|   IBIS Model for tsi109
[IBIS Ver]   3.2
[Disclaimer] This model is subject to change.
   Integrated Device Technology, Inc. ("IDT") hereby grants the
   user of this IBIS model a non-exclusive, nontransferable
   license to use this IBIS model under the following terms. The
   user is granted this license only to use the IBIS model and is
   not granted rights to sell, copy (except as needed to run the
   IBIS model), rent, lease or sub-license the IBIS model in
   whole or in part, or in modified form to anyone. The User may
   modify the IBIS model to suit its specific applications, but
   rights to derivative works and such modifications shall belong
   to IDT. This IBIS model is provided on an AS IS" basis and IDT
   makes absolutely no warranty with respect to the information
   contained herein. IDT DISCLAIMS AND CUSTOMER WAIVES ALL
   WARRANTIES, EXPRESS AND IMPLIED, INCLUDING WARRANTIES OF
   MERCHANTABILITY AND FITNESS FOR A PARTICULAR PURPOSE. THE
   ENTIRE RISK AS TO QUALITY AND PERFORMANCE IS WITH THE USER
   ACCORDINGLY, IN NO EVENT SHALL IDT BE LIABLE FOR ANY DIRECT OR
   INDIRECT DAMAGES, WHETHER IN CONTRACT OR TORT, INCLUDING ANY
   LOST PROFITS OR OTHER INCIDENTAL, CONSEQUENTIAL, EXEMPLARY, OR
   PUNITIVE DAMAGES ARISING OUT OF THE USE OR APPLICATION OF THE
   IBIS model. Further, IDT reserves the right to make changes
   without notice to any product herein to improve reliability,
   function, or design. IDT does not convey any license under
   patent rights or any other intellectual property rights,
   including those of third parties. IDT is not obligated to
   provide maintenance or support for the licensed IBIS model.
[Copyright]   Copyright 2009, Integrated Device Technology, Inc. all
   rights reserved.
[File Name]   tsi109_v3r1_ind.ibs
[File Rev]   3.2
[Date]   03/28/2006
[Notes]
   Revision History
   Rev 1.0
   - 6/17/04 Inital Release. This models is intended for
   evaluation purposes only and does not contain real
   IV/VT curves.  RHB
   Rev 1.1
   - 1/29/2005 First Customer Release. RHB
   Rev 2.0
   -5/24/2005 Regenerated using updated HSPICE models. JMB
   Rev 2.1
   -6/15/2005 Changed models for pins SD_CB[*] to SD_DQ
   from SD_OUT. JMB
   Rev 3.0
   - 02/07/2006  Updated model curves with new simulation data.  RRD
   Rev 3.1
   - 03/28/2006  Add input-only, output-only models.  RRD
   Rev 3.2
   - 09/08/2009 Updated with IDT formatting
[Component] tsi109
[Manufacturer] Integrated Device Technology, Inc.
|   typ   min   max
[Package]
R_pkg   1040.87m   306.00m   1990.00m
L_pkg   5530.5pH   2360.0pH  11100.0pH
C_pkg   2.419pF   1.600pF   4.370pF
[Pin] signal_name   model_name   R_pin   L_pin   C_pin
A1   NC   NC
A2   SD_DQ[56]   SD_DQ   1830.00m  7470.0pH   3.370pF
A3   SD_DQ[60]   SD_DQ   1140.00m  6650.0pH   2.730pF
A4   SD_CLK_N[5]   SD_CLK   1790.00m  6540.0pH   3.670pF
A5   SD_CLK_N[2]   SD_CLK   1690.00m  8020.0pH   2.520pF
A6   SD_CLK_P[2]   SD_CLK   1680.00m  7780.0pH   2.570pF
A7   SD_DQ[34]   SD_DQ   1660.00m  6230.0pH   3.340pF
A8   SD_DQ[38]   SD_DQ   1060.00m  6420.0pH   2.480pF
A9   SD_DQS_P[4]   SD_DQS   1510.00m  7200.0pH   2.400pF
A10   SD_DQS_N[13]   SD_DQS#   1560.00m  6140.0pH   3.180pF
A11   SD_DQ[33]   SD_DQ   1080.00m  6930.0pH   2.450pF
A12   SD_DQ[32]   SD_DQ   1540.00m  6240.0pH   3.020pF
A13   SD_DQ[36]   SD_DQ   1450.00m  5500.0pH   2.910pF
A14   SD_CLK_N[3]   SD_CLK   1530.00m  7950.0pH   2.290pF
A15   SD_CLKFBO_N   SD_OUT   1520.00m  8400.0pH   2.370pF
A16   SD_CLKFBI_P   SD_OUT   1270.00m  4970.0pH   2.770pF
A17   SD_CLK_P[0]   SD_CLK   1520.00m  7380.0pH   2.330pF
A18   SD_DQ[19]   SD_DQ   1030.00m  6390.0pH   2.410pF
A19   SD_DQ[18]   SD_DQ   1000.00m  6450.0pH   2.380pF
A20   SD_DQ[23]   SD_DQ   1020.00m  6410.0pH   2.440pF
A21   SD_DQS_P[2]   SD_DQS   1420.00m  7090.0pH   2.310pF
A22   SD_DQS_N[11]   SD_DQS#   1500.00m  7330.0pH   2.280pF
A23   SD_DQS_P[11]   SD_DQS   1480.00m  7310.0pH   2.390pF
A24   SD_DQ[16]   SD_DQ   1570.00m  6260.0pH   3.010pF
A25   SD_DQ[20]   SD_DQ   1680.00m  6530.0pH   3.200pF
A26   SD_CLK_N[4]   SD_CLK   1700.00m  8530.0pH   2.540pF
A27   SD_CLK_N[1]   SD_CLK   1660.00m  6210.0pH   3.340pF
A28   SD_DQ[3]   SD_DQ   1720.00m  6440.0pH   3.290pF
A29   SD_DQ[2]   SD_DQ   1790.00m  6520.0pH   3.270pF
A30   SD_DQ[6]   SD_DQ   1750.00m  11100.0pH  2.260pF
A31   SD_DQS_N[0]   SD_DQS#   1770.00m  7880.0pH   2.650pF
A32   VSS_IO   GND
B1   SD_DQS_P[16]   SD_DQS   1750.00m  7110.0pH   3.440pF
B2   SD_DQ[57]   SD_DQ   1140.00m  6410.0pH   2.660pF
B3   VSS_IO   GND
B4   NC   NC
B5   SD_CLK_P[5]   SD_CLK   1800.00m  6730.0pH   3.560pF
B6   VSS_IO   GND
B7   SD_DQ[35]   SD_DQ   1590.00m  6010.0pH   3.050pF
B8   SD_DQ[39]   SD_DQ   1030.00m  6400.0pH   2.510pF
B9   VSS_IO   GND
B10   SD_DQS_N[4]   SD_DQS#   1530.00m  7070.0pH   2.410pF
B11   SD_DQS_P[13]   SD_DQS   1560.00m  6020.0pH   3.250pF
B12   VSS_IO   GND
B13   SD_DQ[37]   SD_DQ   964.00m   6360.0pH   2.410pF
B14   SD_CLK_P[3]   SD_CLK   1530.00m  7890.0pH   2.390pF
B15   VSS_IO   GND
B16   SD_CLKFBO_P   SD_OUT   1510.00m  8250.0pH   2.380pF
B17   SD_CLKFBI_N   SD_OUT   1270.00m  5580.0pH   2.860pF
B18   SD_CLK_N[0]   SD_CLK   1500.00m  7590.0pH   2.420pF
B19   VSS_IO   GND
B20   SD_DQ[22]   SD_DQ   1080.00m  7000.0pH   2.540pF
B21   SD_DQS_N[2]   SD_DQS#   1450.00m  7330.0pH   2.340pF
B22   VSS_IO   GND
B23   SD_DQ[17]   SD_DQ   1070.00m  6980.0pH   2.470pF
B24   SD_DQ[21]   SD_DQ   1110.00m  6950.0pH   2.500pF
B25   VSS_IO   GND
B26   SD_CLK_P[4]   SD_CLK   1710.00m  8340.0pH   2.600pF
B27   SD_CLK_P[1]   SD_CLK   1630.00m  6310.0pH   3.440pF
B28   VSS_IO   GND
B29   SD_DQ[7]   SD_DQ   1560.00m  7000.0pH   3.180pF
B30   SD_DQS_P[0]   SD_DQS   1770.00m  8010.0pH   2.710pF
B31   VSS_IO   GND
B32   SD_DQS_N[9]   SD_DQS#   1740.00m  8460.0pH   2.590pF
C1   VSS_IO   GND
C2   SD_DQS_N[16]   SD_DQS#   1730.00m  6400.0pH   3.630pF
C3   SD_DQ[61]   SD_DQ   1200.00m  7870.0pH   2.680pF
C4   VDD_SD   POWER
C5   SD_DQ[54]   SD_DQ   1540.00m  5890.0pH   3.090pF
C6   SD_DQS_N[6]   SD_DQS#   1420.00m  7180.0pH   2.350pF
C7   VDD_SD   POWER
C8   SD_DQ[53]   SD_DQ   1370.00m  5230.0pH   2.990pF
C9   SD_DQ[43]   SD_DQ   1380.00m  5690.0pH   2.850pF
C10   VDD_SD   POWER
C11   SD_DQS_N[5]   SD_DQS#   1220.00m  4990.0pH   2.770pF
C12   SD_DQS_P[14]   SD_DQS   1200.00m  6340.0pH   2.120pF
C13   VDD_SD   POWER
C14   SD_CB[3]   SD_DQ   812.00m   5540.0pH   2.170pF
C15   SD_CB[6]   SD_DQ   789.00m   5680.0pH   2.170pF
C16   VDD_SD   POWER
C17   NC   NC
C18   VDD_SD   POWER
C19   SD_CB[5]   SD_DQ   811.00m   5770.0pH   2.160pF
C20   SD_DQ[26]   SD_DQ   1140.00m  5190.0pH   2.610pF
C21   VDD_SD   POWER
C22   SD_DQS_N[12]   SD_DQS#   1250.00m  5070.0pH   2.780pF
C23   NC   NC
C24   VDD_SD   POWER
C25   SD_DQ[11]   SD_DQ   1030.00m  7050.0pH   2.450pF
C26   SD_DQ[15]   SD_DQ   1330.00m  5270.0pH   2.780pF
C27   VDD_SD   POWER
C28   NC   NC
C29   VDD_SD   POWER
C30   NC   NC
C31   SD_DQS_P[9]   SD_DQS   1720.00m  8030.0pH   2.610pF
C32   SD_DQ[1]   SD_DQ   1780.00m  6690.0pH   3.520pF
D1   SD_DQS_P[7]   SD_DQS   1620.00m  7470.0pH   2.530pF
D2   SD_DQS_N[7]   SD_DQS#   1670.00m  8310.0pH   2.620pF
D3   SD_DQ[62]   SD_DQ   1490.00m  6280.0pH   2.940pF
D4   SD_DQ[51]   SD_DQ   1520.00m  6140.0pH   3.220pF
D5   SD_DQ[55]   SD_DQ   1470.00m  6410.0pH   2.940pF
D6   SD_DQS_P[6]   SD_DQS   1430.00m  7550.0pH   2.330pF
D7   SD_DQS_P[15]   SD_DQS   1320.00m  5410.0pH   2.860pF
D8   SD_DQ[48]   SD_DQ   962.00m   6180.0pH   2.360pF
D9   SD_DQ[52]   SD_DQ   924.00m   6060.0pH   2.270pF
D10   SD_DQ[47]   SD_DQ   1220.00m  5520.0pH   2.700pF
D11   SD_DQS_P[5]   SD_DQS   1220.00m  5110.0pH   2.760pF
D12   SD_DQS_N[14]   SD_DQS#   1200.00m  6280.0pH   2.110pF
D13   SD_DQ[40]   SD_DQ   1150.00m  5330.0pH   2.620pF
D14   SD_DQ[44]   SD_DQ   890.00m   6610.0pH   2.280pF
D15   SD_CB[7]   SD_DQ   670.00m   4800.0pH   2.030pF
D16   SD_DQS_N[8]   SD_DQS#   987.00m   5460.0pH   2.040pF
D17   SD_DQS_N[17]   SD_DQS#   1040.00m  6330.0pH   2.120pF
D18   SD_CB[1]   SD_DQ   1140.00m  5740.0pH   2.500pF
D19   SD_CB[4]   SD_DQ   1120.00m  4840.0pH   2.630pF
D20   SD_DQ[31]   SD_DQ   808.00m   5620.0pH   2.150pF
D21   SD_DQS_P[3]   SD_DQS   1210.00m  5190.0pH   2.790pF
D22   SD_DQS_P[12]   SD_DQS   1250.00m  5470.0pH   2.910pF
D23   SD_DQ[25]   SD_DQ   1230.00m  5240.0pH   2.570pF
D24   SD_DQ[29]   SD_DQ   1230.00m  5420.0pH   2.890pF
D25   SD_DQ[10]   SD_DQ   1020.00m  6620.0pH   2.390pF
D26   SD_DQ[14]   SD_DQ   982.00m   6140.0pH   2.300pF
D27   SD_DQS_N[1]   SD_DQS#   1370.00m  7580.0pH   2.280pF
D28   SD_DQS_P[10]   SD_DQS   1370.00m  5580.0pH   2.950pF
D29   SD_DQ[8]   SD_DQ   1560.00m  6180.0pH   3.040pF
D30   NC   NC
D31   SD_DQ[0]   SD_DQ   1660.00m  6770.0pH   3.180pF
D32   SD_DQ[5]   SD_DQ   1760.00m  6720.0pH   3.460pF
E1   SD_DQ[63]   SD_DQ   1670.00m  6670.0pH   3.160pF
E2   SD_DQ[58]   SD_DQ   1560.00m  6080.0pH   3.120pF
E3   VSS_IO   GND
E4   NC   NC
E5   SD_DQ[50]   SD_DQ   1460.00m  6250.0pH   2.860pF
E6   VSS_IO   GND
E7   SD_DQS_N[15]   SD_DQS#   1320.00m  5370.0pH   2.900pF
E8   SD_DQ[49]   SD_DQ   1150.00m  5080.0pH   2.550pF
E9   VSS_IO   GND
E10   SD_DQ[42]   SD_DQ   777.00m   5310.0pH   2.020pF
E11   SD_DQ[46]   SD_DQ   737.00m   5600.0pH   2.030pF
E12   VSS_IO   GND
E13   SD_DQ[41]   SD_DQ   1010.00m  4810.0pH   2.320pF
E14   SD_DQ[45]   SD_DQ   841.00m   6000.0pH   2.200pF
E15   VSS_IO   GND
E16   SD_DQS_P[8]   SD_DQS   966.00m   5460.0pH   1.970pF
E17   SD_DQS_P[17]   SD_DQS   1050.00m  6280.0pH   2.050pF
E18   SD_CB[0]   SD_DQ   605.00m   4680.0pH   1.880pF
E19   VSS_IO   GND
E20   SD_DQ[30]   SD_DQ   1000.00m  4730.0pH   2.250pF
E21   SD_DQS_N[3]   SD_DQS#   1220.00m  5610.0pH   2.800pF
E22   VSS_IO   GND
E23   SD_DQ[24]   SD_DQ   1110.00m  5050.0pH   2.490pF
E24   SD_DQ[28]   SD_DQ   1230.00m  5670.0pH   2.600pF
E25   VSS_IO   GND
E26   SD_DQS_P[1]   SD_DQS   1370.00m  8240.0pH   2.290pF
E27   SD_DQS_N[10]   SD_DQS#   1350.00m  5470.0pH   3.060pF
E28   VDD_SD   POWER
E29   SD_DQ[13]   SD_DQ   1290.00m  5480.0pH   2.860pF
E30   VSS_IO   GND
E31   SD_DQ[4]   SD_DQ   1560.00m  6390.0pH   3.020pF
E32   CG_PB_SELECT[1]   GEN18_IN   1090.00m  6830.0pH   2.480pF
F1   SD_DQ[59]   SD_DQ   1630.00m  6800.0pH   3.100pF
F2   VSS_IO   GND
F3   NC   NC
F4   NC   NC
F5   NC   NC
F6   NC   NC
F7   SD_ODT[3]   SD_OUT   732.00m   5070.0pH   2.050pF
F8   NC   NC
F9   SD_CSn[1]   SD_OUT   1100.00m  5310.0pH   2.390pF
F10   VDD_SD   POWER
F11   SD_ODT[0]   SD_OUT   592.00m   4280.0pH   1.960pF
F12   NC   NC
F13   VDD_SD   POWER
F14   SD_RASn   SD_OUT   821.00m   4190.0pH   2.230pF
F15   SD_CB[2]   SD_DQ   929.00m   4810.0pH   2.220pF
F16   SD_DLL_TEST[0]   SD_OUT   820.00m   4110.0pH   2.060pF
F17   VDD_SD   POWER
F18   SD_DLL_TEST[1]   SD_OUT   872.00m   4480.0pH   2.170pF
F19   SD_DQ[27]   SD_DQ   647.00m   4860.0pH   1.920pF
F20   SD_A[6]   SD_OUT   919.00m   4540.0pH   2.310pF
F21   VDD_SD   POWER
F22   SD_VREF[1]   POWER   944.00m   4570.0pH   2.260pF
F23   SD_BA[2]   SD_OUT   732.00m   5230.0pH   1.970pF
F24   VDD_SD   POWER
F25   NC   NC
F26   SD_CLKEN[1]   SD_OUT   1140.00m  4900.0pH   2.470pF
F27   VSS_IO   GND
F28   SD_DQ[9]   SD_DQ   1320.00m  5560.0pH   3.000pF
F29   SD_DQ[12]   SD_DQ   1390.00m  5930.0pH   2.860pF
F30   PB_A[33]   PB_IO   1420.00m  5680.0pH   2.910pF
F31   PB_RSTn   GEN18_OUT   981.00m   5810.0pH   2.480pF
F32   CG_REF   GEN18_IN   1050.00m  6430.0pH   2.500pF
G1   HLP_AD[0]   GEN33_IO_tf06it0nn2  1030.00m  6280.0pH   2.530pF
G2   HLP_AD[1]   GEN33_IO_tf06it0nn2  1290.00m  5250.0pH   2.780pF
G3   SD_I2C_CLK   GEN33_OUT_tf12it0pu2 1320.00m  5560.0pH   2.720pF
G4   SD_I2C_SD   GEN33_IO_tf12it0pu2  1200.00m  5350.0pH   2.530pF
G5   HLP_AD[8]   GEN33_IO_tf06it0nn2  1300.00m  5630.0pH   2.620pF
G6   HLP_AD[9]   GEN33_IO_tf06it0nn2  1100.00m  4780.0pH   2.350pF
G7   VSS_IO   GND
G8   SD_ODT[1]   SD_OUT   846.00m   4100.0pH   2.080pF
G9   SD_CSn[3]   SD_OUT   1010.00m  5160.0pH   2.230pF
G10   SD_A[13]   SD_OUT   638.00m   5140.0pH   1.970pF
G11   SD_ODT[2]   SD_OUT   868.00m   4580.0pH   2.050pF
G12   SD_CASn   SD_OUT   821.00m   4410.0pH   2.070pF
G13   SD_WEn   SD_OUT   614.00m   5160.0pH   1.830pF
G14   SD_CSn[0]   SD_OUT   817.00m   4790.0pH   2.120pF
G15   SD_A[10]   SD_OUT   747.00m   3920.0pH   2.090pF
G16   SD_A[0]   SD_OUT   780.00m   4450.0pH   2.130pF
G17   SD_A[2]   SD_OUT   826.00m   4910.0pH   2.100pF
G18   SD_A[1]   SD_OUT   833.00m   4310.0pH   2.050pF
G19   SD_A[4]   SD_OUT   711.00m   6210.0pH   2.120pF
G20   SD_A[9]   SD_OUT   860.00m   5070.0pH   2.160pF
G21   SD_A[8]   SD_OUT   623.00m   5260.0pH   1.830pF
G22   SD_A[11]   SD_OUT   603.00m   4440.0pH   1.830pF
G23   SD_A[14]   SD_OUT   600.00m   4560.0pH   1.860pF
G24   SD_A[15]   SD_OUT   575.00m   4280.0pH   1.840pF
G25   SD_CLKEN[0]   SD_OUT   939.00m   4550.0pH   2.420pF
G26   VDD_SD   POWER
G27   NC   NC
G28   VSS_IO   GND
G29   CG_SD_SELECT[0]   GEN18_IN   814.00m   5410.0pH   2.190pF
G30   NC   NC
G31   VSS_IO   GND
G32   CG_SD_SELECT[1]   GEN18_IN   1370.00m  5250.0pH   2.920pF
H1   HLP_AD[2]   GEN33_IO_tf06it0nn2  996.00m   6180.0pH   2.390pF
H2   HLP_AD[3]   GEN33_IO_tf06it0nn2  1260.00m  5200.0pH   2.750pF
H3   HLP_AD[4]   GEN33_IO_tf06it0nn2  837.00m   5550.0pH   2.280pF
H4   VSS_IO   GND
H5   HLP_AD[5]   GEN33_IO_tf06it0nn2  1130.00m  4790.0pH   2.460pF
H6   HLP_AD[6]   GEN33_IO_tf06it0nn2  870.00m   6390.0pH   2.250pF
H7   HLP_AD[7]   GEN33_IO_tf06it0nn2  853.00m   4190.0pH   2.180pF
H8   NC   NC
H9   VSS_IO   GND
H10   VDD_SD   POWER
H11   VDD_SD   POWER
H12   SD_VREF[0]   POWER   610.00m   3730.0pH   1.830pF
H13   VSS_IO   GND
H14   SD_CSn[2]   SD_OUT   649.00m   8400.0pH   1.970pF
H15   SD_BA[0]   SD_OUT   961.00m   4300.0pH   2.370pF
H16   SD_BA[1]   SD_OUT   736.00m   6940.0pH   2.100pF
H17   VSS_IO   GND
H18   SD_A[3]   SD_OUT   751.00m   4280.0pH   1.920pF
H19   SD_A[5]   SD_OUT   862.00m   5240.0pH   2.080pF
H20   VSS_IO   GND
H21   SD_A[7]   SD_OUT   569.00m   4850.0pH   1.740pF
H22   SD_A[12]   SD_OUT   901.00m   4490.0pH   2.160pF
H23   VDD_SD   POWER
H24   VDD_SD   POWER
H25   VSS_IO   GND
H26   PB_A[34]   PB_IO   960.00m   4820.0pH   2.220pF
H27   VDD_PB   POWER
H28   CG_SD_SELECT[2]   GEN18_IN   684.00m   4920.0pH   2.040pF
H29   CG_PB_SELECT[2]   GEN18_IN   758.00m   5350.0pH   2.080pF
H30   VDD_PB   POWER
H31   CG_PB_CLKO[1]   GEN18_OUT   923.00m   6270.0pH   2.370pF
H32   CG_PB_CLKO[0]   GEN18_OUT   971.00m   6200.0pH   2.410pF
J1   CLKGEN_PLL_AVDD[1]   POWER   491.00m   4760.0pH   3.100pF
J2   CLKGEN_PLL_AVSS[1]   POWER   430.00m   3090.0pH   4.370pF
J3   HLP_AD[10]   GEN33_IO_tf06it0nn2  904.00m   5880.0pH   2.270pF
J4   HLP_AD[11]   GEN33_IO_tf06it0nn2  749.00m   5350.0pH   2.120pF
J5   HLP_AD[12]   GEN33_IO_tf06it0nn2  698.00m   5380.0pH   1.950pF
J6   HLP_AD[13]   GEN33_IO_tf06it0nn2  684.00m   5640.0pH   1.990pF
J7   HLP_AD[14]   GEN33_IO_tf06it0nn2  961.00m   6170.0pH   2.390pF
J8   HLP_AD[15]   GEN33_IO_tf06it0nn2  925.00m   4660.0pH   2.160pF
J9   VDD_PC   POWER
J10   VSS_IO   GND
J11   VDD_SD   POWER
J12   VSS_IO   GND
J13   VDD_SD   POWER
J14   VSS_IO   GND
J15   VDD_SD   POWER
J16   VSS_IO   GND
J17   VDD_SD   POWER
J18   VSS_IO   GND
J19   VDD_SD   POWER
J20   VSS_IO   GND
J21   VDD_SD   POWER
J22   VSS_IO   GND
J23   VDD_SD   POWER
J24   VSS_IO   GND
J25   PB_A[35]   PB_IO   802.00m   4510.0pH   2.010pF
J26   PB_A[10]   PB_IO   903.00m   4680.0pH   2.070pF
J27   PB_A[32]   PB_IO   1000.00m  4980.0pH   2.290pF
J28   PB_A[0]   PB_IO   1040.00m  4790.0pH   2.360pF
J29   PB_TSIZ[2]   PB_IO   839.00m   5660.0pH   2.180pF
J30   NC   NC
J31   CG_PB_SELECT[0]   GEN18_IN   965.00m   6110.0pH   2.420pF
J32   CG_PB_CLKO[2]   GEN18_OUT   977.00m   5900.0pH   2.420pF
K1   HLP_AD[16]   GEN33_IO_tf06it0nn2  1040.00m  6310.0pH   2.480pF
K2   VSS_IO   GND
K3   HLP_AD[17]   GEN33_IO_tf06it0nn2  811.00m   5330.0pH   2.190pF
K4   HLP_AD[18]   GEN33_IO_tf06it0nn2  730.00m   5200.0pH   2.080pF
K5   HLP_AD[19]   GEN33_IO_tf06it0nn2  689.00m   4660.0pH   2.040pF
K6   HLP_AD[20]   GEN33_IO_tf06it0nn2  839.00m   5820.0pH   2.220pF
K7   VSS_IO   GND
K8   HLP_AD[21]   GEN33_IO_tf06it0nn2  923.00m   4970.0pH   2.600pF
K9   VDD_PC   POWER
K10   VDD_PC   POWER
K11   VSS_IO   GND
K12   VDD_SD   POWER
K13   VDD_SD   POWER
K14   VDD_SD   POWER
K15   VDD_SD   POWER
K16   VDD_SD   POWER
K17   VDD_SD   POWER
K18   VDD_SD   POWER
K19   VDD_SD   POWER
K20   VDD_SD   POWER
K21   VDD_SD   POWER
K22   VDD_SD   POWER
K23   VSS_IO   GND
K24   VDD_PB   POWER
K25   PB_TT[3]   PB_IO   1140.00m  5840.0pH   2.280pF
K26   PB_A[8]   PB_IO   739.00m   6390.0pH   2.000pF
K27   PB_A[6]   PB_IO   983.00m   4960.0pH   2.270pF
K28   VSS_IO   GND
K29   CLKGEN_PLL_AVDD[0]   POWER   321.00m   2490.0pH   3.650pF
K30   CLKGEN_PLL_AVSS[0]   POWER   444.00m   4160.0pH   2.900pF
K31   VSS_IO   GND
K32   PB_A[4]   PB_IO   954.00m   5740.0pH   2.420pF
L1   HLP_AD[22]   GEN33_IO_tf06it0nn2  934.00m   5910.0pH   2.300pF
L2   HLP_AD[23]   GEN33_IO_tf06it0nn2  1260.00m  5350.0pH   2.610pF
L3   HLP_AD[24]   GEN33_IO_tf06it0nn2  788.00m   5570.0pH   2.150pF
L4   HLP_AD[25]   GEN33_IO_tf06it0nn2  1030.00m  4620.0pH   2.370pF
L5   VSS_IO   GND
L6   HLP_AD[26]   GEN33_IO_tf06it0nn2  897.00m   4290.0pH   2.260pF
L7   HLP_AD[27]   GEN33_IO_tf06it0nn2  750.00m   6430.0pH   1.890pF
L8   HLP_AD[28]   GEN33_IO_tf06it0nn2  877.00m   4660.0pH   2.060pF
L9   VDD_PC   POWER
L10   VDD_PC   POWER
L11   VSS_IO   GND
L12   VSS_IO   GND
L13   VSS_IO   GND
L14   VSS_IO   GND
L15   VSS_IO   GND
L16   VSS_IO   GND
L17   VSS_IO   GND
L18   VSS_IO   GND
L19   VSS_IO   GND
L20   VSS_IO   GND
L21   VSS_IO   GND
L22   VSS_IO   GND
L23   VDD_PB   POWER
L24   VDD_PB   POWER
L25   PB_AP[4]   PB_IO   753.00m   7660.0pH   2.170pF
L26   PB_TT[1]   PB_IO   315.00m   3030.0pH   2.770pF
L27   VDD_PB   POWER
L28   PB_TT[0]   PB_IO   649.00m   4750.0pH   1.970pF
L29   PB_TT[4]   PB_IO   722.00m   5540.0pH   2.110pF
L30   VDD_PB   POWER
L31   SD_PLL_AVDD   POWER   488.00m   4020.0pH   2.960pF
L32   SD_PLL_AVSS   POWER   386.00m   2570.0pH   4.370pF
M1   HLP_WEn   GEN33_OUT_tf06it0nn2 983.00m   6520.0pH   2.420pF
M2   HLP_CSn[0]   GEN33_OUT_tf06it0nn2 1350.00m  5870.0pH   2.700pF
M3   HLP_CSn[2]   GEN33_OUT_tf06it0nn2 1190.00m  5000.0pH   2.760pF
M4   HLP_CSn[3]   GEN33_OUT_tf06it0nn2 1010.00m  4430.0pH   2.390pF
M5   HLP_LE   GEN33_OUT_tf06it0nn2 1030.00m  5260.0pH   2.300pF
M6   HLP_AD[29]   GEN33_IO_tf06it0nn2  843.00m   3830.0pH   2.240pF
M7   HLP_AD[30]   GEN33_IO_tf06it0nn2  770.00m   5580.0pH   1.970pF
M8   HLP_AD[31]   GEN33_IO_tf06it0nn2  811.00m   4290.0pH   1.990pF
M9   VDD_PC   POWER
M10   VDD_PC   POWER
M11   VSS_IO   GND
M12   VSS   GND
M13   VDD   POWER
M14   VSS   GND
M15   VDD   POWER
M16   VSS   GND
M17   VDD   POWER
M18   VSS   GND
M19   VDD   POWER
M20   VSS   GND
M21   VDD   POWER
M22   VSS_IO   GND
M23   VDD_PB   POWER
M24   VSS_IO   GND
M25   PB_INTn[1]   PB_OUT   1040.00m  5240.0pH   2.930pF
M26   PB_INTn[2]   PB_OUT   890.00m   4640.0pH   2.040pF
M27   PB_INTn[3]   PB_OUT   912.00m   4540.0pH   2.110pF
M28   PB_A[2]   PB_IO   953.00m   4290.0pH   2.310pF
M29   PB_PLL_AVSS   POWER   306.00m   2360.0pH   3.640pF
M30   PB_PLL_AVDD   POWER   1220.00m  5280.0pH   2.510pF
M31   PB_TSIZ[1]   PB_IO   867.00m   5610.0pH   2.270pF
M32   SD_SYSCLK   GEN18_IN   917.00m   5720.0pH   2.310pF
N1   HLP_CSn[1]   GEN33_OUT_tf06it0nn2 978.00m   5920.0pH   2.390pF
N2   VSS_IO   GND
N3   HLP_RDYn   GEN33_IN_it2nn2   752.00m   4880.0pH   2.120pF
N4   HLP_OEn   GEN33_OUT_tf06it0nn2 1090.00m  4980.0pH   2.430pF
N5   GPIO[0]   GEN33_IO_tf06it0nn2  807.00m   5660.0pH   2.090pF
N6   GPIO[1]   GEN33_IO_tf06it0nn2  866.00m   4180.0pH   2.100pF
N7   VSS_IO   GND
N8   U_1_RX   GEN33_IN_it2nn2   627.00m   3560.0pH   1.820pF
N9   VDD_PC   POWER
N10   VDD_PC   POWER
N11   VSS_IO   GND
N12   VDD   POWER
N13   VSS   GND
N14   VDD   POWER
N15   VSS   GND
N16   VDD   POWER
N17   VSS   GND
N18   VDD   POWER
N19   VSS   GND
N20   VDD   POWER
N21   VSS   GND
N22   VSS_IO   GND
N23   VDD_PB   POWER
N24   VDD_PB   POWER
N25   VSS_IO   GND
N26   PB_HITn[1]   PB_IN   946.00m   4810.0pH   2.110pF
N27   PB_BRn[1]   PB_IN   834.00m   4400.0pH   2.030pF
N28   VSS_IO   GND
N29   PB_BRn[0]   PB_IN   676.00m   4760.0pH   1.960pF
N30   PB_AP[2]   PB_IO   823.00m   5440.0pH   2.240pF
N31   VSS_IO   GND
N32   PB_AP[3]   PB_IO   1370.00m  5330.0pH   2.930pF
P1   JTAG_TDO   GEN33_OUT_tf02it0nn2 875.00m   5320.0pH   2.270pF
P2   JTAG_TDI   GEN33_IN_it2pu2   1220.00m  4910.0pH   2.750pF
P3   GPIO[2]   GEN33_IO_tf06it0nn2  730.00m   5170.0pH   2.130pF
P4   VSS_IO   GND
P5   GPIO[3]   GEN33_IO_tf06it0nn2  708.00m   5120.0pH   1.950pF
P6   GPIO[4]   GEN33_IO_tf06it0nn2  876.00m   4260.0pH   2.400pF
P7   GPIO[5]   GEN33_IO_tf06it0nn2  837.00m   6940.0pH   2.070pF
P8   U_0_RX   GEN33_IN_it2nn2   533.00m   3260.0pH   1.750pF
P9   VDD_PC   POWER
P10   VDD_PC   POWER
P11   VSS_IO   GND
P12   VSS   GND
P13   VDD   POWER
P14   VSS   GND
P15   VDD   POWER
P16   VSS   GND
P17   VDD   POWER
P18   VSS   GND
P19   VDD   POWER
P20   VSS   GND
P21   VDD   POWER
P22   VSS_IO   GND
P23   VDD_PB   POWER
P24   VSS_IO   GND
P25   PB_AP[0]   PB_IO   815.00m   4350.0pH   1.940pF
P26   PB_TSIZ[0]   PB_IO   696.00m   5530.0pH   2.040pF
P27   VDD_PB   POWER
P28   PB_TT[2]   PB_IO   659.00m   4860.0pH   1.860pF
P29   PB_QACKn[1]   PB_OUT   741.00m   5010.0pH   2.130pF
P30   VDD_PB   POWER
P31   PB_TBSTn   PB_IO   1230.00m  5310.0pH   2.520pF
P32   PB_SYSCLK   PB_IN   900.00m   6160.0pH   2.320pF
R1   TEST_TM[1]   GEN33_IO_tf02it0nn2  955.00m   5990.0pH   2.330pF
R2   JTAG_TCK   GEN33_IN_it2pu2   1220.00m  5440.0pH   2.730pF
R3   GPIO[6]   GEN33_IO_tf06it0nn2  721.00m   5020.0pH   2.000pF
R4   INT[0]   GEN33_IN_it2nn2   726.00m   5300.0pH   2.040pF
R5   GPIO[7]   GEN33_IO_tf06it0nn2  842.00m   4090.0pH   2.240pF
R6   GPIO[8]   GEN33_IO_tf06it0nn2  833.00m   4360.0pH   2.060pF
R7   GPIO[9]   GEN33_IO_tf06it0nn2  913.00m   4860.0pH   2.080pF
R8   U_1_TX   GEN33_OUT_tf06it0nn2 606.00m   3210.0pH   1.800pF
R9   VDD_PC   POWER
R10   VDD_PC   POWER
R11   VSS_IO   GND
R12   VDD   POWER
R13   VSS   GND
R14   VDD   POWER
R15   VSS   GND
R16   VDD   POWER
R17   VSS   GND
R18   VDD   POWER
R19   VSS   GND
R20   VDD   POWER
R21   VSS   GND
R22   VSS_IO   GND
R23   VDD_PB   POWER
R24   VDD_PB   POWER
R25   PB_QACKn[0]   PB_OUT   647.00m   6420.0pH   1.690pF
R26   PB_A[14]   PB_IO   713.00m   6620.0pH   1.930pF
R27   PB_A[23]   PB_IO   805.00m   4400.0pH   2.000pF
R28   PB_GBLn   PB_IO   924.00m   4510.0pH   2.140pF
R29   PB_A[7]   PB_IO   715.00m   5430.0pH   2.110pF
R30   PB_A[9]   PB_IO   1120.00m  4880.0pH   2.400pF
R31   PB_AP[1]   PB_IO   1200.00m  5610.0pH   2.520pF
R32   PB_HITn[0]   PB_IN   1320.00m  5290.0pH   2.870pF
T1   TEST_TM[3]   GEN33_IO_tf02it0nn2  1310.00m  5340.0pH   2.700pF
T2   VSS_IO   GND
T3   JTAG_TRSTn   GEN33_IN_it2pu2   1120.00m  5010.0pH   2.430pF
T4   GPIO[10]   GEN33_IO_tf06it0nn2  959.00m   5830.0pH   2.390pF
T5   GPIO[11]   GEN33_IO_tf06it0nn2  911.00m   4960.0pH   2.190pF
T6   INT[2]   GEN33_IN_it2nn2   884.00m   7680.0pH   2.250pF
T7   VSS_IO   GND
T8   U_0_TX   GEN33_OUT_tf06it0nn2 494.00m   3200.0pH   1.630pF
T9   VDD_PC   POWER
T10   VDD_PC   POWER
T11   VSS_IO   GND
T12   VSS   GND
T13   VDD   POWER
T14   VSS   GND
T15   VDD   POWER
T16   VSS   GND
T17   VDD   POWER
T18   VSS   GND
T19   VDD   POWER
T20   VSS   GND
T21   VDD   POWER
T22   VSS_IO   GND
T23   VDD_PB   POWER
T24   VSS_IO   GND
T25   PB_A[24]   PB_IO   674.00m   5920.0pH   2.010pF
T26   PB_A[16]   PB_IO   690.00m   5100.0pH   1.950pF
T27   PB_A[3]   PB_IO   856.00m   4060.0pH   2.110pF
T28   VSS_IO   GND
T29   PB_A[1]   PB_IO   714.00m   4980.0pH   1.970pF
T30   PB_A[12]   PB_IO   998.00m   3970.0pH   2.400pF
T31   VSS_IO   GND
T32   PB_INTn[0]   PB_OUT   909.00m   5820.0pH   2.290pF
U1   TEST_TM[2]   GEN33_IO_tf02it0nn2  906.00m   5850.0pH   2.260pF
U2   JTAG_TMS   GEN33_IN_it2pu2   1140.00m  4560.0pH   2.660pF
U3   TEST_ON   GEN33_IN_it2pd2   1030.00m  4240.0pH   2.510pF
U4   INT[1]   GEN33_IN_it2nn2   778.00m   5530.0pH   2.060pF
U5   VSS_IO   GND
U6   GPIO[12]   GEN33_IO_tf06it0nn2  856.00m   4770.0pH   2.110pF
U7   GPIO[13]   GEN33_IO_tf06it0nn2  755.00m   5630.0pH   2.000pF
U8   I2C_SCLK   GEN33_OUT_tf12it0nn2 510.00m   3290.0pH   1.600pF
U9   VDD_PC   POWER
U10   VDD_PC   POWER
U11   VSS_IO   GND
U12   VDD   POWER
U13   VSS   GND
U14   VDD   POWER
U15   VSS   GND
U16   VDD   POWER
U17   VSS   GND
U18   VDD   POWER
U19   VSS   GND
U20   VDD   POWER
U21   VSS   GND
U22   VSS_IO   GND
U23   VDD_PB   POWER
U24   VDD_PB   POWER
U25   VSS_IO   GND
U26   PB_TSn   PB_IO   647.00m   5230.0pH   1.900pF
U27   VDD_PB   POWER
U28   PB_A[21]   PB_IO   891.00m   4330.0pH   2.190pF
U29   PB_DTI[0]   PB_OUT   1050.00m  5060.0pH   2.310pF
U30   VDD_PB   POWER
U31   PB_A[20]   PB_IO   772.00m   5200.0pH   2.180pF
U32   PB_TAn   PB_OUT   1340.00m  5580.0pH   2.720pF
V1   TEST_TM[0]   GEN33_IO_tf02it0nn2  876.00m   5600.0pH   2.220pF
V2   TEST_BIDR_CTL   GEN33_IN_it2pd2   794.00m   5170.0pH   2.170pF
V3   OCN_RSTn   GEN33_IN_it2nn2   785.00m   5110.0pH   2.170pF
V4   GPIO[14]   GEN33_IO_tf06it0nn2  733.00m   6010.0pH   2.010pF
V5   GPIO[15]   GEN33_IO_tf06it0nn2  751.00m   6450.0pH   1.870pF
V6   INT[3]   GEN33_IN_it2nn2   836.00m   3970.0pH   2.080pF
V7   NC   NC
V8   I2C_SD   GEN33_IO_tf12it0nn2  608.00m   3400.0pH   1.860pF
V9   VDD_PC   POWER
V10   VDD_PC   POWER
V11   VSS_IO   GND
V12   VSS   GND
V13   VDD   POWER
V14   VSS   GND
V15   VDD   POWER
V16   VSS   GND
V17   VDD   POWER
V18   VSS   GND
V19   VDD   POWER
V20   VSS   GND
V21   VDD   POWER
V22   VSS_IO   GND
V23   VDD_PB   POWER
V24   VSS_IO   GND
V25   PB_TEAn   PB_OUT   672.00m   6090.0pH   1.860pF
V26   PB_A[22]   PB_IO   836.00m   4100.0pH   2.040pF
V27   PB_A[18]   PB_IO   764.00m   5560.0pH   2.170pF
V28   PB_BGn[1]   PB_OUT   944.00m   4630.0pH   2.130pF
V29   PB_BGn[0]   PB_OUT   739.00m   4930.0pH   2.050pF
V30   PB_A[5]   PB_IO   736.00m   4980.0pH   2.100pF
V31   PB_A[13]   PB_IO   874.00m   5700.0pH   2.290pF
V32   PB_RSTOD   PB_IN   1350.00m  5580.0pH   2.940pF
W1   E_MDIO   GEN33_IO_tf12it0nn2  880.00m   5470.0pH   2.250pF
W2   VSS_IO   GND
W3   E_MDC   GEN33_OUT_tf12it0nn2 1300.00m  5740.0pH   2.690pF
W4   E_1_TCG[9]   GEN33_OUT_tf12it0nn2 665.00m   4520.0pH   1.950pF
W5   E_0_TCG[9]   GEN33_OUT_tf12it0nn2 1180.00m  5540.0pH   2.440pF
W6   E_0_TCG[8]   GEN33_OUT_tf12it0nn2 741.00m   5690.0pH   2.110pF
W7   VSS_IO   GND
W8   E_0_TCG[7]   GEN33_OUT_tf12it0nn2 879.00m   5210.0pH   2.000pF
W9   VDD_PC   POWER
W10   VDD_PC   POWER
W11   VSS_IO   GND
W12   VDD   POWER
W13   VSS   GND
W14   VDD   POWER
W15   VSS   GND
W16   VDD   POWER
W17   VSS   GND
W18   VDD   POWER
W19   VSS   GND
W20   VDD   POWER
W21   VSS   GND
W22   VSS_IO   GND
W23   VDD_PB   POWER
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|**********************DIFF PIN*************************************************
[Diff_pin] inv_pin vdiff tdelay_typ tdelay_min tdelay_max |Signal Comp Signal
A16   B17   .250V   0ns   NA   NA  |SD_CLKFBI_P   SD_CLKFBI_N
B16   A15   .250V   0ns   NA   NA  |SD_CLKFBO_P   SD_CLKFBO_N
A17   B18   .250V   0ns   NA   NA  |SD_CLK_P[0]   SD_CLK_N[0]
B27   A27   .250V   0ns   NA   NA  |SD_CLK_P[1]   SD_CLK_N[1]
A6   A5   .250V   0ns   NA   NA  |SD_CLK_P[2]   SD_CLK_N[2]
B14   A14   .250V   0ns   NA   NA  |SD_CLK_P[3]   SD_CLK_N[3]
B26   A26   .250V   0ns   NA   NA  |SD_CLK_P[4]   SD_CLK_N[4]
B5   A4   .250V   0ns   NA   NA  |SD_CLK_P[5]   SD_CLK_N[5]
B30   A31   .250V   0ns   NA   NA  |SD_DQS_P[0]   SD_DQS_N[0]
E26   D27   .250V   0ns   NA   NA  |SD_DQS_P[1]   SD_DQS_N[1]
A21   B21   .250V   0ns   NA   NA  |SD_DQS_P[2]   SD_DQS_N[2]
D21   E21   .250V   0ns   NA   NA  |SD_DQS_P[3]   SD_DQS_N[3]
A9   B10   .250V   0ns   NA   NA  |SD_DQS_P[4]   SD_DQS_N[4]
D11   C11   .250V   0ns   NA   NA  |SD_DQS_P[5]   SD_DQS_N[5]
D6   C6   .250V   0ns   NA   NA  |SD_DQS_P[6]   SD_DQS_N[6]
D1   D2   .250V   0ns   NA   NA  |SD_DQS_P[7]   SD_DQS_N[7]
E16   D16   .250V   0ns   NA   NA  |SD_DQS_P[8]   SD_DQS_N[8]
C31   B32   .250V   0ns   NA   NA  |SD_DQS_P[9]   SD_DQS_N[9]
D28   E27   .250V   0ns   NA   NA  |SD_DQS_P[10]  SD_DQS_N[10]
A23   A22   .250V   0ns   NA   NA  |SD_DQS_P[11]  SD_DQS_N[11]
D22   C22   .250V   0ns   NA   NA  |SD_DQS_P[12]  SD_DQS_N[12]
B11   A10   .250V   0ns   NA   NA  |SD_DQS_P[13]  SD_DQS_N[13]
C12   D12   .250V   0ns   NA   NA  |SD_DQS_P[14]  SD_DQS_N[14]
D7   E7   .250V   0ns   NA   NA  |SD_DQS_P[15]  SD_DQS_N[15]
B1   C2   .250V   0ns   NA   NA  |SD_DQS_P[16]  SD_DQS_N[16]
E17   D17   .250V   0ns   NA   NA  |SD_DQS_P[17]  SD_DQS_N[17]
|  Pins   are a differential I/O only when DQS# is enabled via MRS
|  If DQS# is disabled, then   (DQS) is a single ended I/O and   is a NC
|   Model Selector
[Model Selector]   SD_DQ
   DQ_odt_75   ODT set to 75ohms
   DQ_odt_150   ODT set to 150ohms
   DQ_no_odt   ODT set to high impedence
[Model Selector]   SD_DQS
   DQS_odt_75   ODT set to 75ohms
   DQS_odt_150   ODT set to 150ohms
   DQS_no_odt   ODT set to high impedence
   DQ_odt_75   DM mode ODT set to 75ohms
   DQ_odt_150   DM mode ODT set to 150ohms
   DQ_no_odt   DM mode ODT set to high impedence
[Model Selector]   SD_DQS#
   DQS_odt_75   ODT set to 75ohms
   DQS_odt_150   ODT set to 150ohms
   DQS_no_odt   ODT set to high impedence
   NC   Set to no connection when in data mask mode
[Model Selector]   PB_IO
   PB_IO_30   Output strength high
   PB_IO_40   Output strength low
[Model Selector]   PB_OUT
   PB_OUT_30   Output strength high
   PB_OUT_40   Output strength low
[Model Selector]   PB_IN
   PB_IN_30   Output strength high
   PB_IN_40   Output strength low
| Models and submodels in the file (31): DQ_odt_75 (I/O), DQ_odt_150 (I/O), DQ_no_odt (I/O), DQS_odt_75 (I/O), DQS_odt_150 (I/O), DQS_no_odt (I/O), PCI_IO (I/O), PCI_OUT (Output), PCI_IN (Input), PB_IO_30 (I/O), PB_OUT_30 (Output), PB_IN_30 (Input), PB_IO_40 (I/O), PB_OUT_40 (Output), PB_IN_40 (Input), GEN18_IO (I/O), GEN18_OUT (Output), GEN18_IN (Input), GEN33_IO_tf12it0nn2 (I/O), GEN33_OUT_tf12it0nn2 (Output), GEN33_IO_tf02it0nn2 (I/O), GEN33_OUT_tf02it0nn2 (Output), GEN33_IO_tf06it0nn2 (I/O), GEN33_OUT_tf06it0nn2 (Output), GEN33_IO_tf12it0pu2 (I/O), GEN33_OUT_tf12it0pu2 (Output), GEN33_IN_it2nn2 (Input), GEN33_IN_it2pd2 (Input), GEN33_IN_it2pu2 (Input), SD_CLK (Output), SD_OUT (Output)
